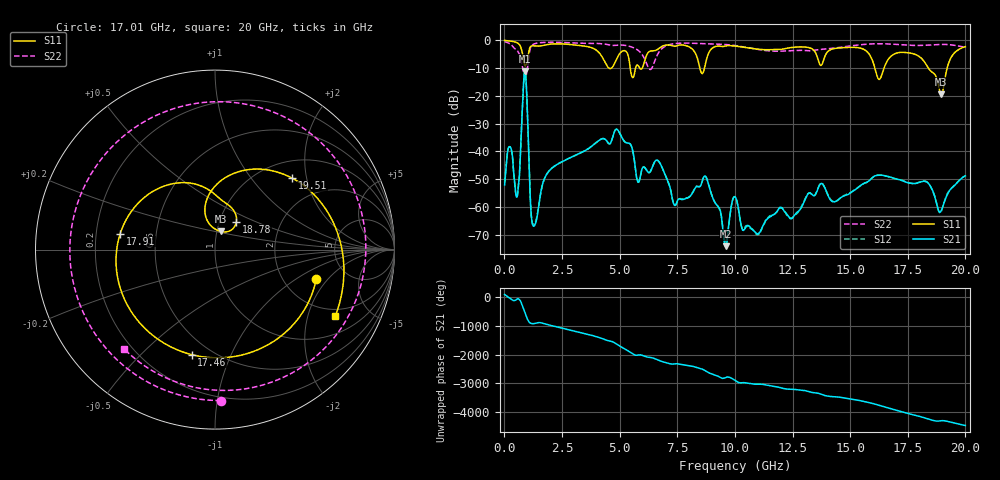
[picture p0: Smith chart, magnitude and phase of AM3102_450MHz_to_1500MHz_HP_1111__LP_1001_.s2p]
!Agilent Technologies,E8364B,MY43040894,A.07.50.67
!Agilent E8364B: A.07.50.67
!Date: Thursday, January 11, 2018 06:50:52
!Correction: S11(Full 2 Port(1,2))
!S21(Full 2 Port(1,2))
!S12(Full 2 Port(1,2))
!S22(Full 2 Port(1,2))
!S2P File: Measurements: S11, S21, S12, S22:
# Hz S  dB  R 50
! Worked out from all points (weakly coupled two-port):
!   1601 points, 10 MHz to 20 GHz, reference 50 ohm
!   highest |S21| = -11.15 dB at 897.1 MHz (marker M1); lowest = -74.1 dB at 9.605 GHz (marker M2)
!   lowest |S11| = -19.5 dB at 18.95 GHz (marker M3), VSWR 1.24, Z = 52.1 + j10.7 ohm
!   |S11| at or under -10 dB: 5.458 GHz to 5.691 GHz (232 MHz wide, 4.16 % of centre); 16.07 GHz to 16.47 GHz (397.2 MHz wide, 2.44 % of centre); 18.39 GHz to 19.21 GHz (815.3 MHz wide, 4.34 % of centre)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
!   |S22| runs from -14.0 to -0.5 dB; largest |S21 - S12| = 0.00058
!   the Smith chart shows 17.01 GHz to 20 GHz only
!   S11 on the Smith chart (normalised r, x): 17.01 GHz: 3.00, -1.53; 17.46 GHz: 0.40, -0.72; 17.91 GHz: 0.30, +0.08; 18.78 GHz: 1.20, +0.39; 19.51 GHz: 1.36, +1.65; 20 GHz: 1.68, -3.01
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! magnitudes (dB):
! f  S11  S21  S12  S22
! 10 MHz  -0.1  -52.1  -51.3  -0.5
! 247.4 MHz  -0.3  -38.4  -38.3  -1.2
! 572.2 MHz  -1.0  -55.5  -55.4  -3.8
! 897.1 MHz  -9.1  -11.1  -11.2  -14.0
! 1.272 GHz  -2.0  -67.0  -66.3  -1.4
! 1.872 GHz  -1.5  -47.8  -47.7  -0.7
! 3.346 GHz  -2.0  -40.4  -40.4  -1.1
! 6.682 GHz  -3.0  -43.5  -43.5  -4.6
! 7.394 GHz  -2.2  -59.5  -59.4  -1.2
! 8.743 GHz  -7.7  -49.2  -49.2  -1.2
! 9.605 GHz  -2.0  -74.1  -72.8  -1.5
! 10.01 GHz  -2.1  -56.3  -56.4  -1.9
! 10.99 GHz  -3.2  -69.8  -70.0  -3.3
! 13.34 GHz  -3.1  -55.5  -55.6  -3.7
! 16.68 GHz  -6.6  -49.1  -49.2  -1.3
! 17.01 GHz  -4.6  -50.0  -50.0  -1.5
! 17.46 GHz  -4.4  -51.2  -51.1  -1.8
! 17.91 GHz  -5.4  -51.4  -51.3  -1.9
! 18.78 GHz  -14.2  -59.7  -59.8  -1.6
! 18.95 GHz  -19.5  -61.4  -61.8  -1.5
! 19.51 GHz  -4.6  -52.4  -52.3  -1.8
! 20 GHz  -2.3  -48.8  -48.8  -2.5
